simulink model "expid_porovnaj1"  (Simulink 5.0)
settings: Solver=ode5  StartTime=0.0  StopTime=500  FixedStep=0.1  RelTol=1e-3

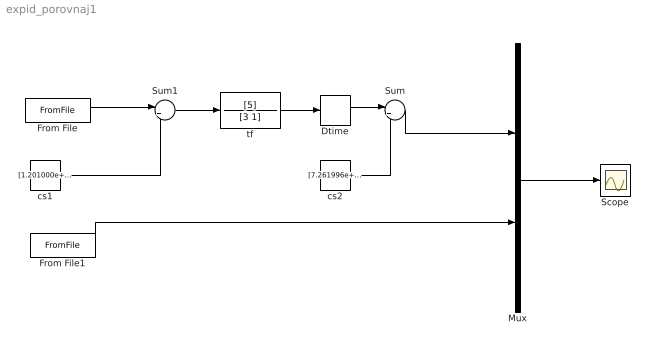
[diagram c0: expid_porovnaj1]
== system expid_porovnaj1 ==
  Dtime : TransportDelay  DelayTime=[1.742935e+000]
  From File : FromFile  FileName=vstup_u.mat  SampleTime=0
  From File1 : FromFile  FileName=vstup_y.mat  SampleTime=0
  Mux : Mux  Inputs=2
  Scope : Scope
  Sum : Sum  Inputs=|++
  Sum1 : Sum  Inputs=|+-
  cs1 : Constant  Value=[1.201000e+001]
  cs2 : Constant  Value=[7.261996e+001]
  tf : TransferFcn  Numerator=[5]  Denominator=[3 1]
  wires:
  cs2/1 -> Sum/2
  Sum/1 -> Mux/1
  From File1/1 -> Mux/2
  From File/1 -> Sum1/1
  Sum1/1 -> tf/1
  cs1/1 -> Sum1/2
  Mux/1 -> Scope/1
  tf/1 -> Dtime/1
  Dtime/1 -> Sum/1
